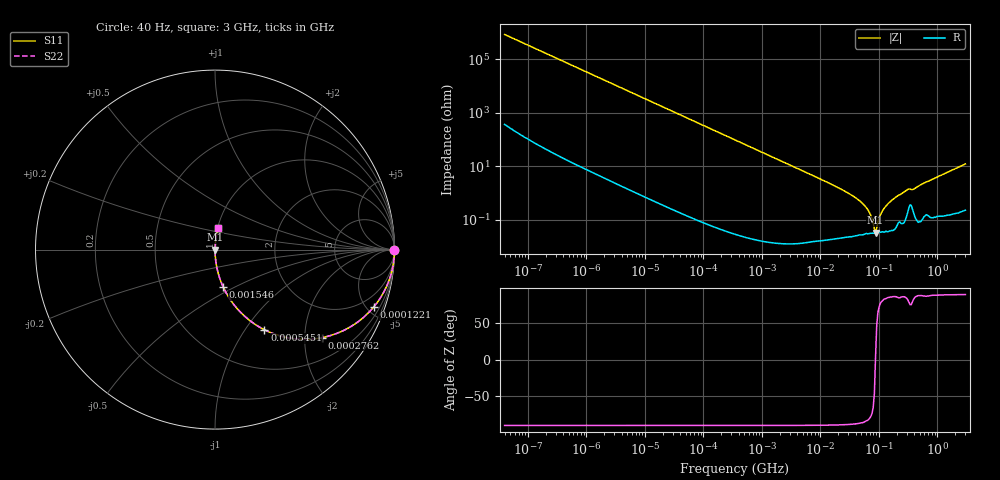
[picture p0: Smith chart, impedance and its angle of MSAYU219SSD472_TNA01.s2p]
! MSAYU219SSD472_TNA01  S-PARAMETER MODEL  ( General Type )
! Model Generated by TAIYO YUDEN Corporation (http://www.ty-top.com)
! Version 2.0
! TAIYO YUDEN Control No. 031016
! Copyright(c) 2003 TAIYO YUDEN CO.,LTD. All Rights Reserved.
! Product Description (link to TY-COMPAS)
! https://ds.yuden.co.jp/TYCOMPAS/or/detail?pn=MSAYU219SSD472KTNA01&u=M
! Products Name : Multilayer Ceramic Capacitors
! Characteristics :
!  Capacitance : 4700 pF , Rated Voltage : 50V
!  Case Size : 2.0 x 1.25 / 0.079 x 0.049 [mm/inch] , Thickness : 0.85 / 0.033 [mm/inch]
!  (Conditions: Temperature = 25 degC , DC Bias Current/Voltage = 0A / 0V)
! External Node Assignments :
!  1  o---| |---o  2
! GND o---------o GND
! Frequency Range : 40Hz  -  3GHz  [ 401 STEP ]
# MHz S RI R 50
! Freq[MHz].  S11 Real  S11 Imag  S21 Real  S21 Imag  S12 Real  S12 Imag  S22 Real  S22 Imag
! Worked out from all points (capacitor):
!   401 points, 40 Hz to 3 GHz, reference 50 ohm
!   read as one part in series: C = 4.74 nF near 44 Hz
!   lowest |Z| = 33 mohm at 87.39 MHz (marker M1)
!   series resonance near 87.19 MHz, so ESL is about 700 pH
!   S11 on the Smith chart (normalised r, x): 40 Hz: open; 122.1 kHz: 1.00, -5.50; 276.2 kHz: 1.00, -2.43; 545.1 kHz: 1.00, -1.23; 1.546 MHz: 1.00, -0.43; 3 GHz: 1.00, +0.24
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4e-05  1 -0.000119  6.6e-08 0.000119  6.6e-08 0.000119  1 -0.000119
0.000834  1 -0.00248  6.72e-06 0.00248  6.72e-06 0.00248  1 -0.00248
0.017386  0.9973 -0.0516  0.00268 0.0516  0.00268 0.0516  0.9973 -0.0516
0.04932  0.9789 -0.1437  0.0211 0.1437  0.0211 0.1437  0.9789 -0.1437
0.122117  0.8832 -0.3211  0.1168 0.3211  0.1168 0.3211  0.8832 -0.3211
0.276155  0.5966 -0.4904  0.4034 0.4904  0.4034 0.4904  0.5966 -0.4904
0.362475  0.4619 -0.4984  0.5381 0.4984  0.5381 0.4984  0.4619 -0.4984
0.545089  0.2752 -0.4464  0.7248 0.4464  0.7248 0.4464  0.2752 -0.4464
1.546262  0.0451 -0.2073  0.9549 0.2073  0.9549 0.2073  0.0451 -0.2073
7.222098  0.00228 -0.0461  0.9977 0.0461  0.9977 0.0461  0.00228 -0.0461
24.56009  0.000372 -0.0125  0.9996 0.0125  0.9996 0.0125  0.000372 -0.0125
46.32945  0.000298 -0.00516  0.9997 0.00516  0.9997 0.00516  0.000298 -0.00516
66.58224  0.000306 -0.00209  0.9997 0.00209  0.9997 0.00209  0.000306 -0.00209
72.90103  0.000313 -0.00139  0.9997 0.00139  0.9997 0.00139  0.000313 -0.00139
79.8195  0.000313 -0.000667  0.9997 0.000667  0.9997 0.000667  0.000313 -0.000667
87.39454  0.00033 1.82e-05  0.9997 -1.82e-05  0.9997 -1.82e-05  0.00033 1.82e-05
91.44753  0.000344 0.000354  0.9997 -0.000354  0.9997 -0.000354  0.000344 0.000354
114.7124  0.00036 0.00211  0.9996 -0.00211  0.9996 -0.00211  0.00036 0.00211
150.5692  0.000398 0.0044  0.9996 -0.0044  0.9996 -0.0044  0.000398 0.0044
297.2015  0.00151 0.0127  0.9985 -0.0127  0.9985 -0.0127  0.00151 0.0127
390.1008  0.00201 0.0137  0.998 -0.0137  0.998 -0.0137  0.00201 0.0137
3000  0.0166 0.1187  0.9834 -0.1187  0.9834 -0.1187  0.0166 0.1187
